ORGANIZATION_BLOCK MAIN:OB1
TITLE=

BEGIN
NETWORK 1
LD I0.0
= Q0.0

NETWORK 2
LD I0.4
O M0.0
A Q0.0
A I0.5
AN I0.3
= M0.0

NETWORK 3
LD M0.0
O I0.6
A I0.1
= Q0.1

NETWORK 4
LD I0.2
= Q0.2

NETWORK 5
LD Q0.0
= Q0.3

END_ORGANIZATION_BLOCK

